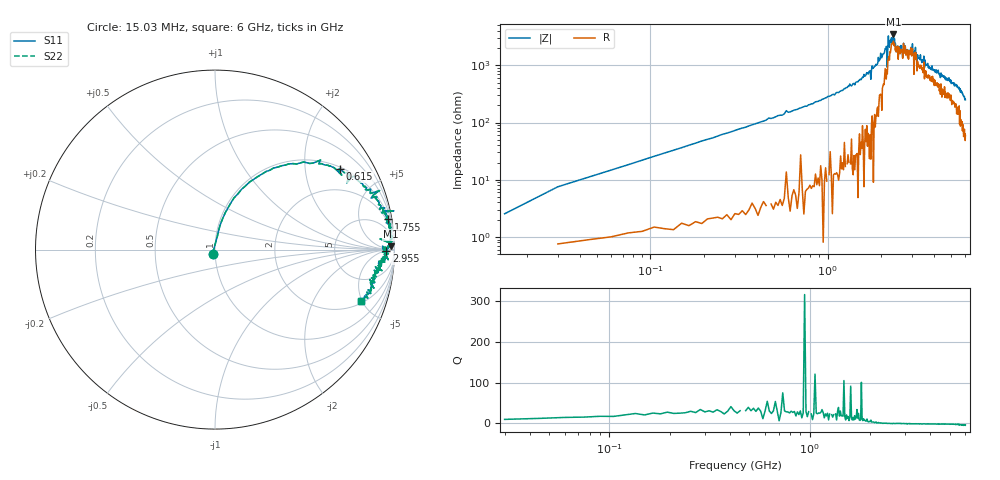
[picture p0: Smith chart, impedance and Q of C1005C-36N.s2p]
!	Network	Analyzer	HP8753E.07.74:	Oct	30	2002	Serial	No.	JP38451487
!	Hewlett-Packard
!	7	Sep	2009	9:05:32
!	Frequency	S11	S21	S12	S22
#	HZ	S	RI	R	50
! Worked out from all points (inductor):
!   400 points, 15.03 MHz to 6 GHz, reference 50 ohm
!   read as one part in series: L = 39.2 nH near 45.03 MHz
!   highest |Z| = 3.46 kohm at 2.355 GHz (marker M1)
!   self-resonance near 2.521 GHz
!   S11 on the Smith chart (normalised r, x): 15.03 MHz: 0.97, -0.04; 615 MHz: 1.06, +3.06; 1.755 GHz: 1, +11; 2.955 GHz: 41, -7; 6 GHz: 2.19, -4.85
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1.502992e7  -0.0137 -0.0228  1.01 0.0228  1.01 0.0228  -0.0137 -0.0228
3.002985e7  0.0129 0.0734  0.987 -0.0734  0.987 -0.0734  0.0129 0.0734
6.00297e7  0.0305 0.142  0.969 -0.142  0.969 -0.142  0.0305 0.142
1.650292e8  0.148 0.336  0.852 -0.336  0.852 -0.336  0.148 0.336
6.150269e8  0.698 0.45  0.302 -0.45  0.302 -0.45  0.698 0.45
1.020025e9  0.881 0.303  0.119 -0.303  0.119 -0.303  0.881 0.303
1.755021e9  0.964 0.168  0.0363 -0.168  0.0363 -0.168  0.964 0.168
1.785021e9  0.977 0.0978  0.0233 -0.0978  0.0233 -0.0978  0.977 0.0978
2.01002e9  0.979 0.0693  0.0205 -0.0693  0.0205 -0.0693  0.979 0.0693
2.160019e9  0.979 0.0422  0.0205 -0.0422  0.0205 -0.0422  0.979 0.0422
2.175019e9  0.92 0.0591  0.0804 -0.0591  0.0804 -0.0591  0.92 0.0591
2.205019e9  0.987 0.0274  0.0128 -0.0274  0.0128 -0.0274  0.987 0.0274
2.235019e9  0.971 0.0366  0.0293 -0.0366  0.0293 -0.0366  0.971 0.0366
2.355018e9  0.978 0.0179  0.0219 -0.0179  0.0219 -0.0179  0.978 0.0179
2.505017e9  0.933 0.0193  0.0672 -0.0193  0.0672 -0.0193  0.933 0.0193
2.535017e9  0.957 -0.0112  0.0435 0.0112  0.0435 0.0112  0.957 -0.0112
2.955015e9  0.954 -0.00763  0.0458 0.00763  0.0458 0.00763  0.954 -0.00763
3.015015e9  0.966 -0.0225  0.0339 0.0225  0.0339 0.0225  0.966 -0.0225
3.195014e9  0.931 -0.0541  0.0687 0.0541  0.0687 0.0541  0.931 -0.0541
4.00501e9  0.926 -0.0901  0.0736 0.0901  0.0736 0.0901  0.926 -0.0901
5.010005e9  0.89 -0.139  0.11 0.139  0.11 0.139  0.89 -0.139
6e9  0.811 -0.288  0.189 0.288  0.189 0.288  0.811 -0.288
